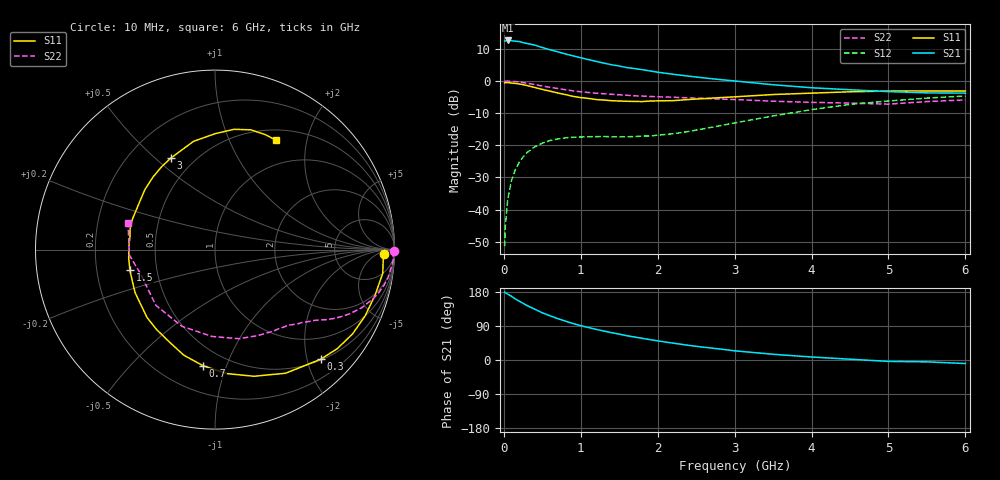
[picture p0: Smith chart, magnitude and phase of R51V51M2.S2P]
! SIEMENS Small Signal Semiconductors
! BFR183
! Si NPN RF Bipolar Junction Transistor in SOT23
! VCE = 1.5 V  IC = 1.2 mA
! Common Emitter S-Parameters:  May  1996
# GHz  S  MA  R  50
!  f  S11  S21  S12  S22
! GHz  MAG  ANG  MAG  ANG  MAG  ANG  MAG  ANG
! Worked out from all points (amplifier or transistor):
!   36 points, 10 MHz to 6 GHz, reference 50 ohm
!   highest |S21| = 12.6 dB at 50 MHz (marker M1)
!   |S21| within 3 dB of that: start of sweep to 617.9 MHz
!   unconditionally stable (mu >= 1): 1.563 GHz to 2.995 GHz
!   at 250 MHz: K = 0.17, MSG = 17.8 dB, |S12| = -23.6 dB
!   at 1.4 GHz: K = 0.91, MSG = 11.2 dB, |S12| = -17.3 dB
!   at 6 GHz: K = 0.96, MSG = 0.4 dB, |S12| = -4.7 dB
!   S11 on the Smith chart (normalised r, x): 10 MHz: 28, -13; 300 MHz: 0.52, -2.25; 700 MHz: 0.37, -0.83; 1.5 GHz: 0.35, -0.10; 3 GHz: 0.37, +0.56; 6 GHz: 0.63, +1.51
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0.01  0.9433 -1.6  4.186 179.3  0.0027 86.7  0.9983 -0.6
0.02  0.9388 -3.2  4.171 177.5  0.0055 86.1  0.99 -1.2
0.05  0.944 -8.0  4.261 174.0  0.0143 85.1  0.9956 -3.2
0.1  0.9272 -15.9  4.215 168.0  0.0285 80.8  0.985 -6.3
0.15  0.9144 -23.8  4.148 161.0  0.0419 75.6  0.9764 -9.3
0.2  0.899 -31.5  4.105 155.2  0.0541 71.7  0.9613 -12.1
0.3  0.8483 -46.1  3.824 143.9  0.0768 63.6  0.923 -17.2
0.4  0.7931 -60.3  3.62 134.2  0.0944 56.5  0.8793 -21.6
0.5  0.7383 -72.9  3.309 124.5  0.1078 50.4  0.8336 -25.3
0.6  0.6943 -84.4  3.056 116.7  0.1186 45.6  0.7964 -28.0
0.7  0.6507 -95.8  2.842 109.3  0.1253 41.5  0.7623 -30.3
0.9  0.575 -116.0  2.453 96.2  0.1333 35.9  0.701 -34.0
1.1  0.5353 -135.0  2.148 85.7  0.1358 32.7  0.6603 -37.3
1.3  0.5055 -151.8  1.894 76.4  0.1369 31.4  0.6317 -40.0
1.5  0.4879 -166.5  1.708 68.3  0.1353 32.2  0.6092 -42.9
1.8  0.4787 172.0  1.496 57.2  0.1388 36.8  0.5819 -47.1
2.2  0.4942 149.8  1.271 44.5  0.1511 44.3  0.5586 -54.5
3  0.566 115.8  1 24.3  0.2224 52.9  0.5148 -74.7
3.5  0.6151 101.2  0.873 15.1  0.2858 50.7  0.4842 -92.0
4.5  0.6785 81.0  0.729 2.1  0.432 37.9  0.4528 -136.8
5.5  0.6991 66.6  0.653 -4.9  0.5412 21.8  0.4781 -176.4
6  0.6981 60.9  0.646 -9.3  0.5835 12.1  0.5076 162.7
